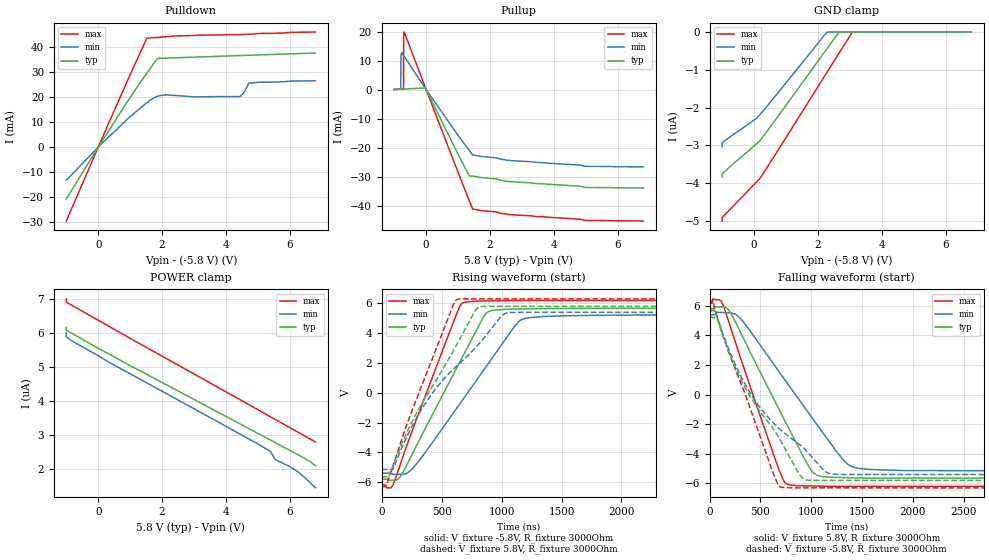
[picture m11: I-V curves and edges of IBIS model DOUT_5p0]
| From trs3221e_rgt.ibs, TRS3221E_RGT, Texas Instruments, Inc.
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[Model]   DOUT_5p0
Model_type   3-state
Polarity   Inverting
Vmeas = 2.5
Vref = 0
Cref = 150pF
Rref = 3000
|variable   typ   min   max
C_comp   6.70pF   5.86pF   7.51pF
|C_pullup   6.79pF   6.08pF   7.38pF
|C_pulldown   6.54pF   5.54pF   7.65pF
[Voltage Range]   11.6   10.8   12.6
[Temperature Range]   27   110   -40
[Pullup Reference]   5.8   5.4   6.3
[Pulldown Reference]   -5.8   -5.4   -6.3
[Power Clamp Reference]   5.8   5.4   6.3
[GND Clamp Reference]   -5.8   -5.4   -6.3
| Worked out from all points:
|   slope of the pulldown table from 0 to 1.74 V, typ, clamps not added: 52 ohm
|   slope of the pullup table from 0 to 1.74 V, typ, clamps not added: 57.4 ohm
|   falling waveform, V_fixture 5.8V, R_fixture 3000Ohm: 20-80 % time 506ns typ, 660ns min, 371ns max; typ from 5.8 V to -5.64 V
|   rising waveform, V_fixture -5.8V, R_fixture 3000Ohm: 20-80 % time 444ns typ, 560ns min, 351ns max; typ from -5.8 V to 5.67 V
|   rising waveform, V_fixture 5.8V, R_fixture 3000Ohm: 20-80 % time 474ns typ, 607ns min, 352ns max; typ from -5.64 V to 5.8 V
|   falling waveform, V_fixture -5.8V, R_fixture 3000Ohm: 20-80 % time 569ns typ, 679ns min, 402ns max; typ from 5.67 V to -5.8 V
[Pulldown]
|	Voltage   I(typ)   I(min)   I(max)
-1V       -20.69mA   -13.21mA   -29.48mA
121.7mV   2.419mA    1.551mA    3.562mA
975.3mV   19.36mA    11.94mA    28.26mA
1.525V    29.58mA    17.81mA    43.51mA
1.856V    35.45mA    20.31mA    43.81mA
2.156V    35.58mA    20.85mA    44.08mA
3.033V    35.96mA    20.07mA    44.64mA
4.428V    36.57mA    20.23mA    44.94mA
4.464V    36.58mA    20.4mA     44.96mA
4.586V    36.64mA    22.27mA    45.02mA
4.713V    36.69mA    25.62mA    45.08mA
6.8V      37.6mA     26.51mA    45.97mA
[GND Clamp]
|   Voltage   I(typ)   I(min)   I(max)
-1V       -3.829uA   -3.033uA   -4.999uA
-1V       -3.77uA    -2.976uA   -4.939uA
-1V       -3.759uA   -2.965uA   -4.928uA
-1V       -3.742uA   -2.949uA   -4.912uA
-999.7mV  -3.742uA   -2.934uA   -4.909uA
-947.9mV  -3.704uA   -2.894uA   -4.86uA
18.77mV   -2.999uA   -2.317uA   -4.016uA
256.3mV   -2.793uA   -2.113uA   -3.784uA
2.275V    -449nA     -6.698nA   -1.074uA
2.651V    -9.95nA    0A         -570.8nA
3.071V    0A         0A         -11.67nA
6.8V      0A         0A         0A
[Pullup]
|	Voltage   I(typ)   I(min)   I(max)
-1V       58.5uA     47.9uA     71.7uA
-800mV    163.2uA    219.8uA    162.4uA
-787.3mV  169.9uA    11.17mA    168.1uA
-778.7mV  174.4uA    12.51mA    172.1uA
-709.6mV  210.6uA    11.87mA    203.4uA
-706.5mV  212.2uA    11.82mA    1.796mA
-705.2mV  212.9uA    11.8mA     14.41mA
-703.4mV  213.9uA    11.77mA    18.21mA
-686.7mV  222.6uA    11.49mA    19.85mA
-24.92mV  569.4uA    410.9uA    731.3uA
1.455V    -29.77mA   -22.5mA    -41.14mA
6.8V      -33.87mA   -26.6mA    -45.24mA
[POWER Clamp]
|   Voltage   I(typ)   I(min)   I(max)
-1V       6.156uA    5.99uA     6.993uA
-1V       6.096uA    5.932uA    6.931uA
-1V       6.077uA    5.912uA    6.913uA
-999.8mV  6.077uA    5.883uA    6.897uA
-868.4mV  6.007uA    5.785uA    6.828uA
813.9mV   5.131uA    4.894uA    5.938uA
5.361V    2.874uA    2.544uA    3.556uA
5.565V    2.772uA    2.278uA    3.45uA
5.981V    2.565uA    2.09uA     3.231uA
6.244V    2.434uA    1.934uA    3.093uA
6.632V    2.226uA    1.612uA    2.89uA
6.8V      2.106uA    1.459uA    2.802uA
[Ramp]
R_load = 3000
|   typ   min   max
dV/dt_r   6.88151/4.4365e-07   6.37009/5.58783e-07   7.49789/3.50473e-07
dV/dt_f   6.86701/5.05661e-07   6.32828/6.60407e-07   7.49816/3.70613e-07
[Falling Waveform]
V_fixture = 5.8V
V_fixture_min = 5.4V
V_fixture_max = 6.3V
R_fixture = 3000Ohm
C_fixture = 0F
|   Time   V(typ)   V(min)   V(max)
0s        5.8V       5.4V       6.3V
128.7ns   5.921V     5.547V     6.104V
187.5ns   5.71V      5.528V     4.934V
299.1ns   4.273V     5.175V     2.58V
660.4ns   -686.8mV   1.775V     -4.654V
761.6ns   -2.051V    798.5mV    -6.044V
1.025us   -5.316V    -1.724V    -6.175V
1.3us     -5.602V    -4.278V    -6.191V
1.423us   -5.622V    -4.911V    -6.192V
4us       -5.645V    -5.148V    -6.197V
[Rising Waveform]
V_fixture = -5.8V
V_fixture_min = -5.4V
V_fixture_max = -6.3V
R_fixture = 3000Ohm
C_fixture = 0F
|   Time   V(typ)   V(min)   V(max)
0s        -5.8V      -5.399V    -6.3V
85.81ns   -5.886V    -5.455V    -6.302V
162.8ns   -5.521V    -5.475V    -4.623V
288ns     -3.588V    -4.8V      -1.831V
632.1ns   1.763V     -963.6mV   5.443V
680.8ns   2.51V      -410.2mV   6.05V
882.5ns   5.41V      1.887V     6.159V
1.116us   5.612V     4.534V     6.186V
1.199us   5.624V     4.99V      6.187V
4us       5.67V      5.217V     6.197V
[Rising Waveform]
V_fixture = 5.8V
V_fixture_min = 5.4V
V_fixture_max = 6.3V
R_fixture = 3000Ohm
C_fixture = 0F
|   Time   V(typ)   V(min)   V(max)
0s        -5.645V    -5.148V    -6.197V
39.22ns   -5.644V    -5.146V    -6.218V
59.01ns   -5.663V    -5.146V    -5.731V
91.67ns   -4.945V    -5.154V    -4.958V
341.8ns   -640.1mV   -992.1mV   634.4mV
629.9ns   3.295V     1.831V     6.264V
798.8ns   5.678V     3.167V     6.298V
1.002us   5.797V     5.165V     6.298V
1.076us   5.797V     5.385V     6.298V
4us       5.8V       5.4V       6.3V
[Falling Waveform]
|Gnd
V_fixture = -5.8V
V_fixture_min = -5.4V
V_fixture_max = -6.3V
R_fixture = 3000Ohm
C_fixture = 0F
|   Time   V(typ)   V(min)   V(max)
0s        5.67V      5.217V     6.197V
29.22ns   5.666V     5.215V     6.354V
69.12ns   5.279V     5.347V     5.378V
199.9ns   2.688V     2.876V     2.647V
341.8ns   566.7mV    796.4mV    172.8mV
625ns     -2.297V    -1.894V    -5.297V
697.2ns   -3.091V    -2.373V    -6.253V
931.9ns   -5.733V    -3.643V    -6.298V
1.223us   -5.797V    -5.382V    -6.298V
4us       -5.8V      -5.399V    -6.3V
